PROGRAM MAIN_CM

VAR CONSTANT
	cInitCounting 	: ST_CM_RainflowCounting_InitPars 		:= ( 	nBins					:= cRfRangeBins, 				// Number of stress bins
																	fMinStress				:= cRfRangeMin,			// Min stress range, i.e. zero or min modulated amplitude of signal beeing counted
																	fMaxStress				:= cRfRangeMax, 			// Max stress range, i.e. greater or equal max modulated amplitude of signal beeing counted
																	nBinsMean				:= cRfMeanBins, 			// Number of mean stress bins
																	fMinMean				:= cRfMeanMin, 			// Lower limit of mean stress
																	fMaxMean				:= cRfMeanMax, 			// Upper limit of mean stress
																	nChannels				:= 1);					// Number of channels
	                                                                                                                        
	cInitMeanStrCorr : ST_CM_MeanStressCorrection_InitPars	:= (	eMeanStressCorrection 	:= cMSCType,                    
																	nBins					:= cRfRangeBins, 				// Number of stress bins
																	fBinWidth				:= cBinWidthRange,			// Bin width of stress ranges w.r.t. fMinStress and fMaxStress of RainflowCounting
																	nBinsMean				:= cRfMeanBins, 			// Number of mean stress bins
																	fBinWidthMean			:= cBinWidthMean, 		// Width of mean stress bins w.r.t. fMinMean and fMaxMean of RainflowCounting
																	fUTS					:= cUTS,				// Ultimate tensile strength of material
																	nChannels				:= 1);					// Number of channels
																	                                                        
	cInitMinersRule : ST_CM_MinersRule_InitPars 			:= ( 	nBins					:= cRfRangeBins,				// First dimension of Output generated by FB_CMA_RainflowCounting.
																	nBinsMean				:= cRfMeanBins,			// Second dimension of Output generated by FB_CMA_RainflowCounting.
																	fDamage					:= cBaseDamage,			// Constant damage at startup
																	nCycles					:= nBaseCycles,			// Constant number of Cycles at startup
																	nChannels				:= 1);					// Number of channels
END_VAR

VAR	
	fbCounting			: FB_CMA_RainflowCounting :=(stInitPars := cInitCounting, nOwnID := eID_RainflowCounting, aDestIDs := [eID_MeanStressCorrection, eID_MinersRule_RFC, eID_Sink_RFC], nResultBuffers := 6);
	fbMeanStressCorr	: FB_CMA_MeanStressCorrection := (stInitPars := cInitMeanStrCorr, nOwnID := eID_MeanStressCorrection, aDestIDs := [eID_MinersRule_MSC, eID_Sink_MSC], nResultBuffers := 5);
	fbMinersRule_RFC	: FB_CMA_MinersRule := (stInitPars := cInitMinersRule, nOwnID := eID_MinersRule_RFC, aDestIDs := [eID_Sink_MR_RFC]);
	fbMinersRule_MSC	: FB_CMA_MinersRule := (stInitPars := cInitMinersRule, nOwnID := eID_MinersRule_MSC, aDestIDs := [eID_Sink_MR_MSC]);
	
	// Sink data
	fbSink_RFC			: FB_CMA_Sink := (nOwnID := eID_Sink_RFC);
	fbSink_MSC			: FB_CMA_Sink := (nOwnID := eID_Sink_MSC);
	
	// Rainflow Counting results
	aRFCResult			: ARRAY[0..cRfRangeBins+1] OF ARRAY[0..cRfMeanBins+1] OF ULINT;	// 0: underflow bin; N+1: overflow bin
	aRFCResult_Mean		: ARRAY[0..cRfMeanBins+1] OF ULINT;
	aRFCResult_Range	: ARRAY[0..cRfRangeBins+1] OF ULINT;
	nRFCResult_Cycles	: ULINT;
	
	// MeanStress correction results
	aMSCResult			: ARRAY[0..cRfRangeBins+1] OF ARRAY[0..cRfMeanBins+1] OF ULINT;	// 0: underflow bin; N+1: overflow bin
	aMSCResult_Mean		: ARRAY[0..cRfMeanBins+1] OF ULINT;
	aMSCResult_Range	: ARRAY[0..cRfRangeBins+1] OF ULINT;
	
	// Configuration args
	isConfigured_MR		: BOOL := FALSE;
	configureArgs 		: ARRAY[0..(cRfRangeBins+1)] OF LREAL;
	configureRFC		: LREAL := cRfRangeMax * (cRfRangeBins + 1) / (cRfRangeMax - cRfRangeMin);	// unused.
	bReset				: BOOL := FALSE;
	
	isConfigure_MSC 	: BOOL := TRUE;
	eCorrection			: E_CM_MeanStressCorrection := E_CM_MeanStressCorrection.eCM_Goodman;
	
	// Transition points of Woehler curve
	fTP, fTP_UTS		: LREAL;
	
	// Status and error handling
	bCalculate			: BOOL;
	fbErrHist			: FB_HRErrHist; 		// error monitoring
	
	// local vars
	hr					: HRESULT;	
	i,n,m				: UDINT;
END_VAR

// Configure MinersRule
Configure();

// Call Algorithms
CallAlgorithms();

// Collect results
CollectResults();

METHOD CallAlgorithms : BOOL
VAR_INPUT
END_VAR
// Call RainflowCounting
fbCounting.Call();
IF fbCounting.bError THEN
	fbErrHist.AddError(bErr:=TRUE, hrErrCode:=fbCounting.hrErrorCode, sErrSource:='MAIN_CM.fbCounting'); // error monitoring
	// ToDo: if error
END_IF

// Mean stress correction
fbMeanStressCorr.Call();
IF fbMeanStressCorr.bError THEN
	fbErrHist.AddError(bErr:=TRUE, hrErrCode:=fbMeanStressCorr.hrErrorCode, sErrSource:='MAIN_CM.fbMeanStressCorr'); // error monitoring
	// ToDo: if error
END_IF

// Call Miners Rule
fbMinersRule_RFC.Call();
IF fbMinersRule_RFC.bError THEN
	fbErrHist.AddError(bErr:=TRUE, hrErrCode:=fbMinersRule_RFC.hrErrorCode, sErrSource:='MAIN_CM.fbMinersRule_RFC.Call'); // error monitoring
	// ToDo: if error
END_IF

// Reset damage control (set persistent damage to zero)
IF bReset THEN
	fbMinersRule_RFC.ResetData();
	IF fbMinersRule_RFC.bError THEN
		fbErrHist.AddError(bErr:=TRUE, hrErrCode:=fbMinersRule_RFC.hrErrorCode, sErrSource:='MAIN_CM.fbMinersRule_RFC.Reset'); // error monitoring
		// ToDo: if error
	END_IF
END_IF

// Call Miners Rule
fbMinersRule_MSC.Call();
IF fbMinersRule_MSC.bError THEN
	fbErrHist.AddError(bErr:=TRUE, hrErrCode:=fbMinersRule_MSC.hrErrorCode, sErrSource:='MAIN_CM.fbMinersRule_MSC.Call'); // error monitoring
	// ToDo: if error
END_IF

// Reset damage control (set persistent damage to zero)
IF bReset THEN
	fbMinersRule_MSC.ResetData();
	IF fbMinersRule_MSC.bError THEN
		fbErrHist.AddError(bErr:=TRUE, hrErrCode:=fbMinersRule_MSC.hrErrorCode, sErrSource:='MAIN_CM.fbMinersRule_MSC.Reset'); // error monitoring
		// ToDo: if error
	END_IF
END_IF
END_METHOD

METHOD CollectResults : BOOL
VAR_INPUT
END_VAR
(* Plain RainflowCounting without Mean-stress correction *)

// Push results to sink
fbSink_RFC.Output2DStd(	pDataOut 		:= ADR(aRFCResult), 
						nDataOutSize 	:= SIZEOF(aRFCResult), 
						eElementType 	:= eMA_TypeCode_UINT64,
						nOptionPars 	:= 0 ,			
						bNewResult		=> bCalculate );// Push results to sink

IF fbSink_RFC.bError THEN
	fbErrHist.AddError(bErr:=TRUE, hrErrCode:=fbSink_RFC.hrErrorCode, sErrSource:='MAIN.fbSink_RFC'); // error monitoring
	// ToDo: if error
END_IF

// Transpose copy for scope
IF bCalculate THEN
	MEMSET(ADR(aRFCResult_Mean), 0, (cRfMeanBins + 1) * SIZEOF(ULINT));
	MEMSET(ADR(aRFCResult_Range), 0, (cRfRangeBins + 1) * SIZEOF(ULINT));
	nRFCResult_Cycles := 0;
	// Sum up range/mean bins
	FOR n := 0 TO cRfRangeBins + 1 DO
		FOR m := 0 TO cRfMeanBins + 1 DO
			aRFCResult_Mean[m] := aRFCResult_Mean[m] + aRFCResult[n][m];
			aRFCResult_Range[n] := aRFCResult_Range[n] + aRFCResult[n][m];
			nRFCResult_Cycles := nRFCResult_Cycles + aRFCResult[n][m];
		END_FOR
	END_FOR
END_IF

(* RainflowCounting with Mean-stress correction *)

// Push results to sink
fbSink_MSC.Output2DStd(	pDataOut 		:= ADR(aMSCResult), 
						nDataOutSize 	:= SIZEOF(aMSCResult), 
						eElementType 	:= eMA_TypeCode_UINT64,
						nOptionPars 	:= 0 ,			
						bNewResult		=> bCalculate );// Push results to sink

IF fbSink_MSC.bError THEN
	fbErrHist.AddError(bErr:=TRUE, hrErrCode:=fbSink_MSC.hrErrorCode, sErrSource:='MAIN.fbSink_MSC'); // error monitoring
	// ToDo: if error
END_IF

// Transpose copy for scope
IF bCalculate THEN
	MEMSET(ADR(aMSCResult_Mean), 0, (cRfMeanBins + 1) * SIZEOF(ULINT));
	MEMSET(ADR(aMSCResult_Range), 0, (cRfRangeBins + 1) * SIZEOF(ULINT));
	// Sum up range/mean bins
	FOR n := 0 TO cRfRangeBins + 1 DO
		FOR m := 0 TO cRfMeanBins + 1 DO
			aMSCResult_Mean[m] := aMSCResult_Mean[m] + aMSCResult[n][m];
			aMSCResult_Range[n] := aMSCResult_Range[n] + aMSCResult[n][m];
		END_FOR
	END_FOR
END_IF
END_METHOD

METHOD Configure : BOOL
VAR_INPUT
END_VAR
IF NOT isConfigured_MR THEN
	// Set user defined values, e.g. same limit for all bins
	//	FOR i:=0 TO (cRfRangeBins + 1) DO
	//	 	configureArgs[i] := cCyclesToFailure;
	//	END_FOR

	// Calculate Woehler curve for damage accumulation
	hr := F_CM_CalculateWoehlerCurve(fSRI := cSRI, fUTS := cUTS, bUseUTSCorrection := cUseUTSCorrection,
									 fK1 := cK1, fK2 := cK2, nNC1 := cNC1, nNC2 := cNC2, fRRatio := cRRatio,
									 fStepsize := cBinWidthRange, nCurveLength := cRfRangeBins + 2, pCurve := ADR(configureArgs));
	 // Fatigue transition point
	fTP := cSRI * EXPT(ULINT_TO_LREAL(cNC2), -1.0 / cK1);
	// Transition point UTS correction
	fTP_UTS := cSRI * EXPT(ULINT_TO_LREAL(cNC1), -1.0 / cK1);

	// Configure algorithm
	IF SUCCEEDED(hr) THEN
		hr := fbMinersRule_RFC.Configure(ADR(configureArgs), SIZEOF(configureArgs));
		IF fbMinersRule_RFC.bError THEN
			fbErrHist.AddError(bErr:=TRUE, hrErrCode:=fbMinersRule_RFC.hrErrorCode, sErrSource:='MAIN_CM.fbMinersRule_RFC'); // error monitoring
			// ToDo: if error
		END_IF
	END_IF
	IF SUCCEEDED(hr) THEN
		hr := fbMinersRule_MSC.Configure(ADR(configureArgs), SIZEOF(configureArgs));
		IF fbMinersRule_MSC.bError THEN
			fbErrHist.AddError(bErr:=TRUE, hrErrCode:=fbMinersRule_MSC.hrErrorCode, sErrSource:='MAIN_CM.fbMinersRule_MSC'); // error monitoring
			// ToDo: if error
		END_IF
	END_IF
	
	// Update status
	IF SUCCEEDED(hr) THEN
		isConfigured_MR := FALSE;
	END_IF
END_IF

IF NOT isConfigure_MSC THEN
	// Configure algorithm
	hr := fbMeanStressCorr.Configure(ADR(eCorrection), SIZEOF(eCorrection));
	IF fbMeanStressCorr.bError THEN
		fbErrHist.AddError(bErr:=TRUE, hrErrCode:=fbMeanStressCorr.hrErrorCode, sErrSource:='MAIN_CM.fbMeanStressCorr'); // error monitoring
		// ToDo: if error
	END_IF
	
	// Update status
	IF SUCCEEDED(hr) THEN
		isConfigured_MR := FALSE;
	END_IF
END_IF
END_METHOD

END_PROGRAM
